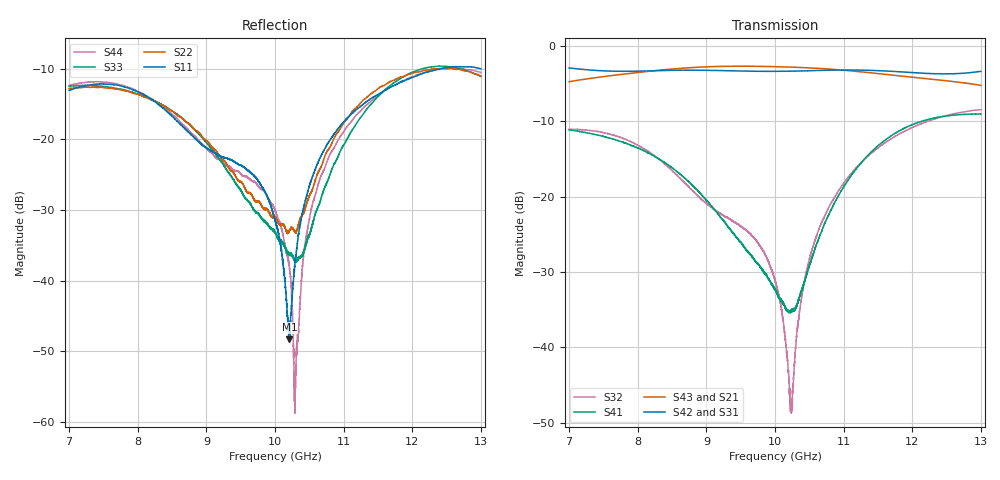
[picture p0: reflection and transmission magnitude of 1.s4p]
# GHZ S DB R 50.00000
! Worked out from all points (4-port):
!   6401 points, 7 GHz to 13 GHz, reference 50 ohm
!   strongest paths, dB at 7 GHz, 8.5 GHz, 10 GHz, 11.5 GHz, 13 GHz:
!     S42: -2.9, -3.3, -3.4, -3.3, -3.4
!     S43: -4.8, -3.1, -2.8, -3.7, -5.3
!     S31: -3.0, -3.3, -3.5, -3.4, -3.5
!     S21: -4.7, -3.1, -2.8, -3.8, -5.4
!     S41: -11.2, -16.2, -32.3, -13.3, -9.0
!     S32: -11.1, -16.6, -31.1, -13.5, -8.5
!   lowest |S11| = -48.3 dB at 10.21 GHz (marker M1), VSWR 1.01, Z = 50.2 + j0.333 ohm
!   |S11| at or under -10 dB: start of sweep to 12.41 GHz; 12.99324 GHz to 12.99757 GHz (4.328 MHz wide, 0.0333 % of centre); 12.99872 GHz to end of sweep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
7  -13.06 168.7  -4.71 -115.4  -3.01 157.2  -11.16 -116.6
   -4.71 -115.4  -12.80 149.7  -11.07 53.5  -2.95 -35.5
   -3.01 157.2  -11.07 53.5  -12.46 148.2  -4.77 53.6
   -11.16 -116.6  -2.94 -35.5  -4.76 53.6  -12.38 147.6
9.699063  -25.18 -13.4  -2.75 163.3  -3.47 74.5  -28.33 -149.4
          -2.74 163.3  -28.58 88.7  -25.49 76.5  -3.38 -53.7
          -3.46 74.5  -25.49 76.5  -30.09 77.3  -2.72 37.7
          -28.33 -149.3  -3.38 -53.7  -2.72 37.7  -26.05 85.0
10.21  -48.29 59.6  -2.85 147.4  -3.46 58.9  -35.30 -87.5
       -2.85 147.4  -32.90 -0.3  -45.76 113.8  -3.37 -57.1
       -3.46 58.9  -45.45 117.0  -36.06 10.5  -2.83 34.2
       -35.33 -87.5  -3.37 -57.1  -2.83 34.2  -38.21 73.2
10.30094  -36.48 118.4  -2.88 144.6  -3.44 56.0  -34.78 -61.1
          -2.88 144.6  -33.08 -20.4  -40.03 -134.3  -3.36 -57.8
          -3.45 56.1  -40.04 -135.6  -37.15 -15.6  -2.86 33.6
          -34.83 -60.9  -3.35 -57.8  -2.86 33.6  -53.09 -28.0
10.4875  -27.02 124.9  -2.96 138.8  -3.40 50.1  -29.53 -29.2
         -2.96 138.7  -28.32 -66.0  -28.86 -120.1  -3.31 -59.3
         -3.40 50.1  -28.84 -120.1  -33.72 -65.0  -2.93 32.3
         -29.47 -28.7  -3.31 -59.3  -2.93 32.3  -32.01 -104.3
10.89062  -18.86 109.6  -3.23 126.4  -3.31 36.8  -20.44 -22.9
          -3.23 126.3  -19.32 -97.6  -19.75 -123.3  -3.23 -63.0
          -3.31 36.8  -19.75 -123.2  -22.98 -96.4  -3.16 29.7
          -20.46 -22.9  -3.23 -63.0  -3.16 29.7  -20.66 -104.8
13  -10.02 6.7  -5.36 65.9  -3.53 -29.1  -9.04 -109.3
    -5.36 66.0  -11.05 -83.5  -8.48 -157.0  -3.39 -78.9
    -3.54 -29.1  -8.48 -157.1  -11.10 -87.4  -5.27 20.2
    -9.04 -109.3  -3.40 -79.0  -5.26 20.2  -10.54 -82.5
